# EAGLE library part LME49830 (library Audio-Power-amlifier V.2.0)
The LME49830 is a high fidelity audio power amplifier input stage designed for demanding consumer and proaudio applications. Amplifier output power may be scaled by changing the supply voltage and number of output devices. The LME49830 is capable of driving an output stage in excess of 300 W single-ended into an 8Ω load in the presence of 10% high line headroom and 20% supply regulation. The LME49830 includes internal thermal shut down circuitry that activates when the LME49830 die temperature exceeds 150°C. The LME49830 has a mute function that mutes the input drive signal and forces the amplifier output to a quiescent state. The LME49830 has high drive current, 56mA typical, and high output voltage swing for maximum flexibility in output stage choice. With a bias voltage range up to 16V the LME49830 can be used to drive MOSFET output stages using a wide selection of MOSFETs.
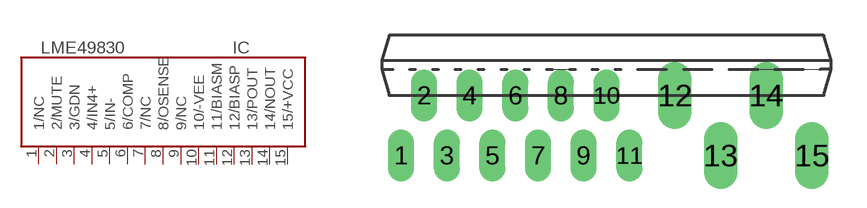
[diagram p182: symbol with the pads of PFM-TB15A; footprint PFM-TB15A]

Designator prefix IC

## LME49830  [PFM-TB15A]
1  1/NC  nc
2  2/MUTE  in
3  3/GDN  pwr
4  4/IN4+  in
5  5/IN-  in
6  6/COMP  in
7  7/NC  nc
8  8/OSENSE  out
9  9/NC  nc
10  10/-VEE  pwr
11  11/BIASM
12  12/BIASP
13  13/POUT  out
14  14/NOUT  out
15  15/+VCC  pwr

## Footprint PFM-TB15A (pad centres in mm)
www.ti.com/audio
drill 0.6 long: 1 -8.685,-2.54; 2 -7.72,-0.001; 3 -6.754,-2.54; 4 -5.789,-0.001; 5 -4.824,-2.541; 6 -3.859,-0.001; 7 -2.894,-2.541; 8 -1.929,-0.001; 9 -0.964,-2.541; 10 0.001,-0.001; 11 0.966,-2.541
drill 0.6 pad 1.422 long: 12 2.896,-0.001; 13 4.826,-2.541; 14 6.756,-0.001; 15 8.686,-2.542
